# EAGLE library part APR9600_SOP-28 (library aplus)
SINGLE-CHIP VOICE RECORDING & PLAYBACK DEVICE FOR SINGLE 60 SECOND # Created by SCRIPT exported from Ultra Librarian Gold 5.3.88 Copyright © 1999-2010 # Tanvir Mohammed, Premier Farnell 2013-04-24 alf@cadsoft.de
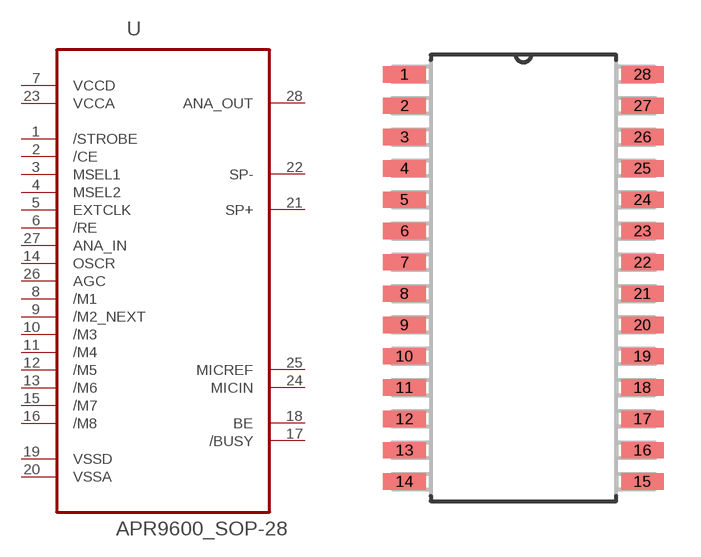
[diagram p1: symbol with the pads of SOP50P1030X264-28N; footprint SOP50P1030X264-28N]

Designator prefix U

## APR9600_SOP-28 (MPN: APR9600_SOP-28; OC_FARNELL: unknown; OC_NEWARK: unknown; PACKAGE: SOP-28; SUPPLIER: APLUS INTEGRATED CIRCUITS INC)  [SOP50P1030X264-28N]
1  /STROBE  in
2  /CE  in
3  MSEL1  in
4  MSEL2  in
5  EXTCLK  in
6  /RE  in
7  VCCD  pwr
8  /M1  in
9  /M2_NEXT  in
10  /M3  in
11  /M4  in
12  /M5  in
13  /M6  in
14  OSCR  in
15  /M7  in
16  /M8  in
17  /BUSY  in
18  BE  in
19  VSSD  pas
20  VSSA  pas
21  SP+  out
22  SP-  out
23  VCCA  pwr
24  MICIN  in
25  MICREF  in
26  AGC  in
27  ANA_IN  in
28  ANA_OUT  out

## Footprint SOP50P1030X264-28N (pad centres in mm)
# Created by Ultra Librarian Gold 5.3.88 Copyright © 1999-2010 # Tanvir Mohammed, Premier Farnell
smd 1.727 x 0.66: 1 -4.826,8.255; 2 -4.826,6.985; 3 -4.826,5.715; 4 -4.826,4.445; 5 -4.826,3.175; 6 -4.826,1.905; 7 -4.826,0.635; 8 -4.826,-0.635; 9 -4.826,-1.905; 10 -4.826,-3.175; 11 -4.826,-4.445; 12 -4.826,-5.715; 13 -4.826,-6.985; 14 -4.826,-8.255; 15 4.826,-8.255; 16 4.826,-6.985; 17 4.826,-5.715; 18 4.826,-4.445; 19 4.826,-3.175; 20 4.826,-1.905; 21 4.826,-0.635; 22 4.826,0.635; 23 4.826,1.905; 24 4.826,3.175; 25 4.826,4.445; 26 4.826,5.715; 27 4.826,6.985; 28 4.826,8.255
